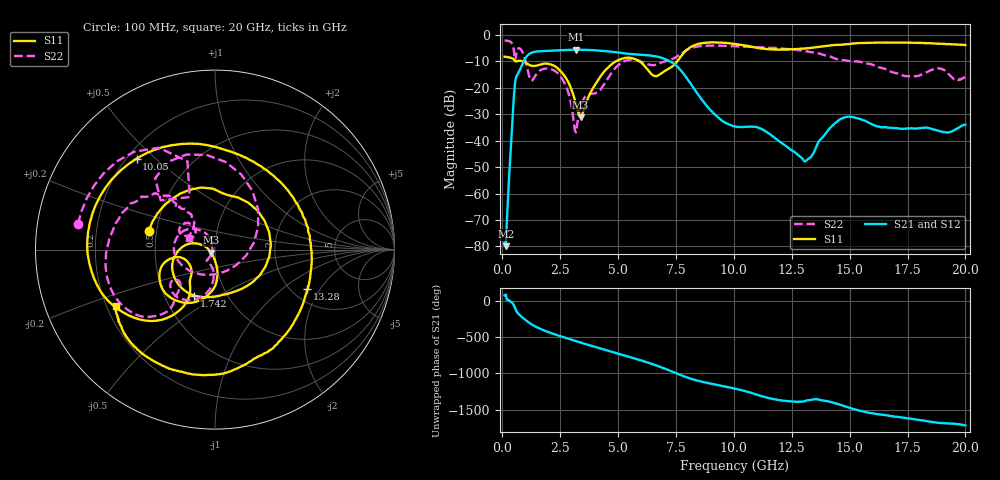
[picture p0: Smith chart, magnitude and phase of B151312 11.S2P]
!  2-Port S-parameters saved by WinCal
! VAR MeasName=S-Parameters (CALIBRATED_DATA) read from VNA (N5244A)
! VAR MeasDate=12/8/2015 5:44:28 PM
! VAR NAME=B151312 11
! VAR FILENAME=B151312 11.S2P
! VAR DATE=12/8/2015 5:44:28 PM
! VAR PHYS_PORTS=1,2
# Hz S DB R 50
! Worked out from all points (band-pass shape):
!   401 points, 100 MHz to 20 GHz, reference 50 ohm
!   highest |S21| = -5.68 dB at 3.184 GHz (marker M1); lowest = -79.9 dB at 149.8 MHz (marker M2)
!   |S21| within 3 dB of the highest: 1.016 GHz to 6.854 GHz (5.839 GHz wide, 148 % of centre)
!   lowest |S11| = -31.3 dB at 3.384 GHz (marker M3), VSWR 1.06, Z = 47.8 - j1.55 ohm
!   |S11| at or under -10 dB: 558.9 MHz to 636.9 MHz (78.03 MHz wide, 13.1 % of centre); 857.3 MHz to 4.918 GHz (4.061 GHz wide, 141 % of centre); 5.909 GHz to 7.563 GHz (1.654 GHz wide, 24.5 % of centre)
!   |S22| runs from -37.0 to -2.2 dB; largest |S21 - S12| = 0.0016
!   S11 on the Smith chart (normalised r, x): 100 MHz: 0.45, +0.11; 1.742 GHz: 0.70, -0.39; 10.05 GHz: 0.24, +0.44; 13.28 GHz: 2.42, -1.55; 20 GHz: 0.24, -0.25
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1e8  -8.33 164.2  -78.54 78.5  -82.59 175.8  -2.19 169.3
1.4975e8  -8.37 156.1  -79.89 88.9  -87.49 7.2  -2.23 163.9
5.975e8  -10.13 75.8  -15.98 -132.3  -15.98 -132.3  -7.78 137.9
1.095e9  -11.11 -39.8  -7.80 74.8  -7.80 74.8  -13.22 9.6
1.74175e9  -11.04 -114.2  -6.20 -38.7  -6.20 -38.7  -13.04 -171.0
2.5875e9  -14.46 177.2  -5.87 -134.3  -5.88 -134.3  -16.76 130.1
3.1845e9  -26.15 165.5  -5.68 165.7  -5.68 165.7  -36.98 -164.9
3.3835e9  -31.28 -143.5  -5.70 146.1  -5.69 146.1  -27.23 -126.2
3.43325e9  -30.51 -125.5  -5.70 141.3  -5.70 141.3  -25.83 -126.8
4.08e9  -17.92 -83.9  -5.94 79.3  -5.93 79.3  -21.90 -116.3
4.876e9  -10.21 -109.8  -6.59 4.3  -6.59 4.3  -12.64 -99.3
5.871e9  -9.81 -160.1  -7.53 -88.1  -7.51 -88.2  -9.82 -140.1
6.7665e9  -15.22 -139.2  -8.46 176.2  -8.47 176.1  -10.92 -133.1
8.10975e9  -4.82 -137.4  -18.21 9.8  -18.19 9.8  -5.20 -137.1
9.00525e9  -2.94 177.2  -28.67 -61.1  -28.67 -61.6  -4.14 -161.3
1.005e10  -3.49 130.7  -34.69 -130.3  -34.74 -130.3  -4.34 -178.9
1.1443e10  -5.44 66.3  -36.89 104.9  -36.93 104.9  -4.91 164.1
1.328375e10  -5.03 -23.1  -46.52 72.5  -46.51 73.0  -6.56 140.3
1.338325e10  -4.95 -26.9  -45.48 79.2  -45.40 79.8  -6.69 138.4
1.47265e10  -3.74 -71.5  -31.41 -6.8  -31.34 -6.6  -9.66 131.4
1.67165e10  -2.99 -113.5  -35.15 -144.2  -34.99 -144.5  -13.68 126.6
2e10  -3.93 -150.4  -34.01 81.7  -34.01 80.8  -15.96 155.5
